ORGANIZATION_BLOCK MAIN:OB1
TITLE=

BEGIN
NETWORK 1
LD I0.0
= Q0.0

NETWORK 2
LD I1.0
A I0.1
= M0.2

NETWORK 3
LD I0.2
O M0.1
A M0.2
A I0.1
= M0.1

NETWORK 4
LD M0.1
O I0.3
A I0.6
A M0.2
= Q0.1

NETWORK 5
LD I0.7
A M0.2
= Q0.2

NETWORK 6
LD I0.5
A M0.2
= Q0.3

NETWORK 7
LD I0.4
AN I0.6
A M0.2
= Q0.4

NETWORK 8
LD Q0.0
= Q0.5

NETWORK 9
LD M0.1
= Q0.6

END_ORGANIZATION_BLOCK

